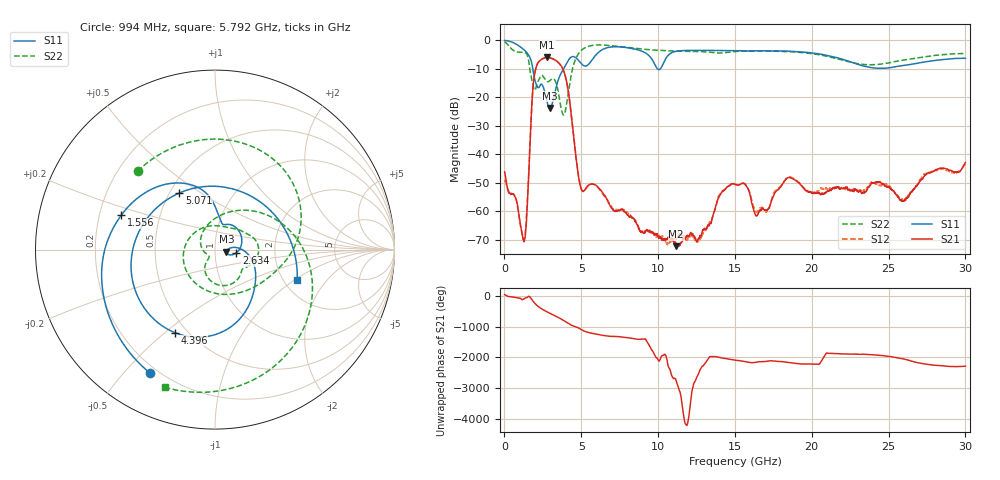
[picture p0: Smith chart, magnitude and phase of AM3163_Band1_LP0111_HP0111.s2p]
!Agilent Technologies,E8364B,MY43040894,A.07.50.67
!Agilent E8364B: A.07.50.67
!Date: Thursday, August 20, 2020 11:18:45
!Correction: S11(Full 2 Port(1,2))
!S21(Full 2 Port(1,2))
!S12(Full 2 Port(1,2))
!S22(Full 2 Port(1,2))
!S2P File: Measurements: S11, S21, S12, S22:
# Hz S  dB  R 50
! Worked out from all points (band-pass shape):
!   3201 points, 10 MHz to 30 GHz, reference 50 ohm
!   highest |S21| = -6.06 dB at 2.784 GHz (marker M1); lowest = -72.2 dB at 11.18 GHz (marker M2)
!   |S21| within 3 dB of the highest: 2.088 GHz to 3.698 GHz (1.61 GHz wide, 55.6 % of centre)
!   lowest |S11| = -23.7 dB at 2.953 GHz (marker M3), VSWR 1.14, Z = 56.8 - j1.31 ohm
!   |S11| at or under -10 dB: 1.845 GHz to 3.854 GHz (2.009 GHz wide, 70.5 % of centre); 9.949 GHz to 10.15 GHz (203 MHz wide, 2.02 % of centre)
!   |S22| runs from -26.2 to -0.5 dB; largest |S21 - S12| = 0.0046
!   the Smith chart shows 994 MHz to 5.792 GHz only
!   S11 on the Smith chart (normalised r, x): 994 MHz: 0.17, -0.59; 1.556 GHz: 0.29, +0.16; 2.634 GHz: 1.27, -0.05; 4.396 GHz: 0.43, -0.54; 5.071 GHz: 0.56, +0.41; 5.792 GHz: 2.37, -1.04
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1e7  -0.08 -7.8  -46.11 48.2  -48.91 65.5  -0.54 -22.2
5.34825e8  -0.77 -62.5  -53.89 -30.7  -53.92 -30.9  -3.39 -143.2
9.940469e8  -2.18 -117.6  -62.84 -72.7  -63.47 -69.4  -4.24 134.7
1.303319e9  -3.50 -158.9  -70.36 -80.2  -68.92 165.6  -4.24 77.3
1.556359e9  -5.09 159.8  -50.12 -9.6  -49.42 18.0  -6.61 8.0
1.949978e9  -13.20 87.5  -12.31 136.3  -12.32 136.3  -17.37 106.8
2.634125e9  -18.42 -8.7  -6.16 -119.3  -6.17 -119.3  -13.68 -26.8
2.784075e9  -21.91 -20.0  -6.06 -159.3  -6.08 -159.4  -14.51 -34.3
2.952769e9  -23.74 -10.2  -6.18 157.7  -6.20 157.6  -14.17 -42.5
3.852469e9  -10.02 -46.6  -10.76 -78.5  -10.78 -78.4  -26.23 -137.6
4.396038e9  -5.78 -115.9  -28.48 119.7  -28.43 119.8  -10.81 49.4
5.014581e9  -8.27 134.0  -52.45 -17.5  -52.25 -17.7  -3.52 -43.4
5.070812e9  -8.57 122.3  -52.95 -32.9  -52.78 -33.3  -3.26 -49.3
5.792447e9  -6.24 -20.1  -50.56 -145.1  -50.41 -145.9  -1.76 -110.0
7.516872e9  -2.34 -170.4  -59.46 110.9  -59.43 110.1  -2.23 158.0
1.000979e10  -10.27 86.3  -68.90 68.0  -69.02 -52.9  -3.55 60.3
1.118128e10  -3.87 59.1  -72.22 111.7  -69.60 26.4  -3.82 18.8
1.5005e10  -3.65 -72.0  -50.54 68.8  -50.51 69.3  -3.96 -90.3
2.000958e10  -4.44 163.6  -53.43 -57.0  -53.26 -55.5  -4.71 136.7
2.276491e10  -8.05 59.9  -52.46 -91.9  -52.10 -99.7  -8.00 20.8
2.500479e10  -9.70 -62.2  -51.34 -168.8  -51.05 -168.1  -7.97 -92.3
3e10  -6.35 104.6  -42.87 -127.9  -43.34 -127.3  -4.65 102.6
